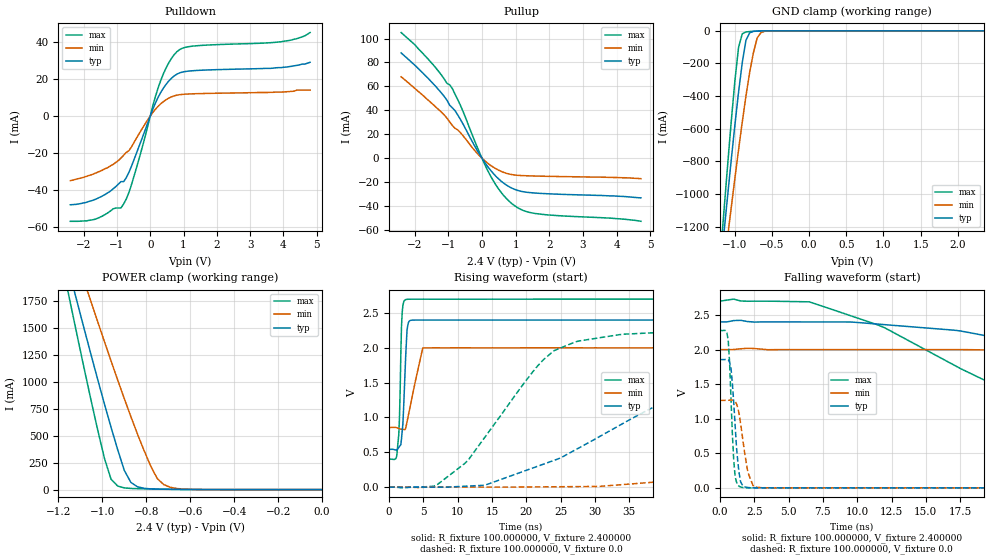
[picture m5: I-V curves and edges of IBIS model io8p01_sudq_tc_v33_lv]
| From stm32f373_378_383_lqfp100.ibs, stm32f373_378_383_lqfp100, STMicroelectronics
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|   Model io8p01_sudq_tc_v33_lv
[Model]  io8p01_sudq_tc_v33_lv
Model_type I/O
Polarity   Non-Inverting
Enable   Active-Low
Vinl =   0.720000V
Vinh =   1.680000V
Vmeas =  1.200000V
Cref =   50.000000pF
Rref =   100.000000M
Vref =   0.0V
C_comp   1.373400pF   1.288200pF   1.481900pF
[Temperature Range]   25.000000   0.125000k   -40.000000
[Pullup Reference]   2.400000V   2.000000V   2.700000V
[Pulldown Reference]   0.0V   0.0V   0.0V
[POWER Clamp Reference]   2.400000V   2.000000V   2.700000V
[GND Clamp Reference]   0.0V   0.0V   0.0V
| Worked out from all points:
|   slope of the pulldown table from 0 to 0.36 V, typ, clamps not added: 25.7 ohm
|   slope of the pullup table from 0 to 0.36 V, typ, clamps not added: 26.8 ohm
|   GND clamp passes 1 mA (typ) near -0.67 V on its own axis
|   POWER clamp passes 1 mA (typ) near -0.60 V on its own axis
|   rising waveform, R_fixture 100.000000, V_fixture 2.400000: 20-80 % time 482ps typ, 1.47ns min, 337ps max; typ from 0.542 V to 2.4 V
|   rising waveform, R_fixture 100.000000, V_fixture 0.0: 20-80 % time 22.2ns typ, 64.5ns min, 10.4ns max; typ from 0 V to 1.85 V
|   falling waveform, R_fixture 100.000000, V_fixture 2.400000: 20-80 % time 28.3ns typ, 66.2ns min, 14.6ns max; typ from 2.4 V to 0.542 V
|   falling waveform, R_fixture 100.000000, V_fixture 0.0: 20-80 % time 389ps typ, 568ps min, 290ps max; typ from 1.85 V to 0 V
[Pulldown]
|Voltage   I(typ)   I(min)   I(max)
-2.4V     -47.8mA    -34.8mA    -56.7mA
-1.68V    -45.1mA    -31mA      -55.7mA
-1.12V    -39.3mA    -26.1mA    -50.05mA
-800mV    -35.33mA   -21.13mA   -47.42mA
-640mV    -30.33mA   -18.65mA   -41.16mA
-480mV    -23.12mA   -14mA      -31.94mA
240mV     10.22mA    5.339mA    15.38mA
480mV     17.22mA    8.864mA    26.1mA
800mV     22.59mA    11.27mA    34.68mA
1.36V     24.54mA    12.05mA    37.84mA
3.92V     26.1mA     12.9mA     40mA
4.8V      29mA       14mA       45mA
[Pullup]
|Voltage   I(typ)   I(min)   I(max)
-2.4V     88mA       68mA       105mA
-2V       77.9mA     58.5mA     95mA
-1.36V    59.6mA     42.5mA     75.1mA
-880mV    42.12mA    27.44mA    58.22mA
-560mV    28.45mA    18.75mA    39mA
-160mV    7.44mA     4.66mA     10.64mA
160mV     -6.607mA   -3.947mA   -9.704mA
480mV     -16.91mA   -9.806mA   -25.1mA
880mV     -24.9mA    -13.63mA   -37.75mA
1.2V      -27.87mA   -14.5mA    -43.37mA
1.6V      -29.13mA   -14.89mA   -46.24mA
4.72V     -33.1mA    -17.1mA    -52.7mA
[GND_clamp]
|Voltage   I(typ)   I(min)   I(max)
-2.4V     -7.358A    -6.372A    -8.78A
-1.2V     -1.489A    -1.65A     -1.416A
-1.15V    -1.254A    -1.461A    -1.124A
-1.1V     -1.024A    -1.273A    -838.2mA
-1.05V    -797.6mA   -1.088A    -563.1mA
-950mV    -374.6mA   -728.7mA   -100.8mA
-900mV    -194.3mA   -557.9mA   -18.01mA
-850mV    -56.94mA   -397.4mA   -7.08mA
-750mV    -3.582mA   -133.8mA   -2.771mA
-700mV    -1.516mA   -44.7mA    -1.516mA
-600mV    -235.4uA   -2.939mA   -209.5uA
2.35V     0A         0A         0A
[POWER_clamp]
|Voltage   I(typ)   I(min)   I(max)
-2.4V     9.979A     9.967A     9.901A
-1.17V    2.182A     2.481A     1.978A
-1.14V    1.945A     2.294A     1.683A
-1.11V    1.71A      2.108A     1.391A
-1.08V    1.476A     1.923A     1.102A
-1.05V    1.245A     1.739A     819.9mA
-960mV    578.2mA    1.196A     96.06mA
-900mV    179.5mA    846.7mA    16.04mA
-870mV    67.18mA    678.8mA    10.82mA
-780mV    6.749mA    219.9mA    5.853mA
-720mV    3.355mA    46.34mA    3.808mA
0V        0A         0A         0A
[Ramp]
| variable   typ   min   max
dV/dt_r  1.11324/22.19804n   0.75702/64.45118n   1.36566/10.36042n
dV/dt_f  1.11491/28.25132n   0.68552/66.25244n   1.37972/14.56637n
R_load = 100.000000
[Rising Waveform]
R_fixture= 100.000000
V_fixture= 2.400000
V_fixture_min= 2.000000
V_fixture_max= 2.700000
|time   V(typ)   V(min)   V(max)
0s        541.6mV    855mV      400.5mV
1.101ns   529.4mV    853mV      447.2mV
1.502ns   582.7mV    838.2mV    994.7mV
1.802ns   699.1mV    831mV      2.319V
1.902ns   805mV      829.9mV    2.51V
2.402ns   1.861V     840.9mV    2.693V
2.603ns   2.251V     937mV      2.697V
2.803ns   2.361V     1.033V     2.699V
4.905ns   2.4V       1.999V     2.699V
49.85ns   2.4V       2V         2.7V
[Rising Waveform]
R_fixture= 100.000000
V_fixture= 0.0
V_fixture_min= 0.0
V_fixture_max= 0.0
|time   V(typ)   V(min)   V(max)
0s        804.5pV    13.47nV    619.4pV
7.007ns   -400.8uV   -241.5uV   34.47mV
11.51ns   14.35mV    -205.9uV   386.8mV
21.02ns   277.4mV    2.191mV    1.667V
24.02ns   383.8mV    4.367mV    1.959V
34.03ns   911.8mV    35.85mV    2.196V
47.55ns   1.541V     139.3mV    2.258V
64.56ns   1.771V     320.8mV    2.271V
139.1ns   1.856V     1.127V     2.276V
249.2ns   1.855V     1.266V     2.276V
[Falling Waveform]
R_fixture= 100.000000
V_fixture= 2.400000
V_fixture_min= 2.000000
V_fixture_max= 2.700000
|time   V(typ)   V(min)   V(max)
0s        2.4V       2V         2.7V
6.507ns   2.4V       2V         2.691V
17.52ns   2.27V      2V         1.727V
27.03ns   1.852V     1.973V     879.4mV
36.04ns   1.464V     1.914V     534.3mV
53.05ns   873.3mV    1.702V     439.5mV
69.07ns   654mV      1.497V     410.3mV
105.1ns   565.8mV    1.136V     399.9mV
152.2ns   545.1mV    929.7mV    400.5mV
249.2ns   541.6mV    855mV      400.5mV
[Falling Waveform]
R_fixture= 100.000000
V_fixture= 0.0
V_fixture_min= 0.0
V_fixture_max= 0.0
|time   V(typ)   V(min)   V(max)
0s        1.855V     1.266V     2.276V
600.6ps   1.852V     1.267V     2.134V
800.8ps   1.732V     1.271V     1.293V
1.001ns   1.236V     1.265V     402.6mV
1.101ns   910.1mV    1.251V     165.3mV
1.301ns   370.5mV    1.154V     40.75mV
1.602ns   51.19mV    789.6mV    6.524mV
2.102ns   3.8mV      186.5mV    555.5uV
2.903ns   239.4uV    4.493mV    318.7uV
49.85ns   804.5pV    13.47nV    619.4pV
